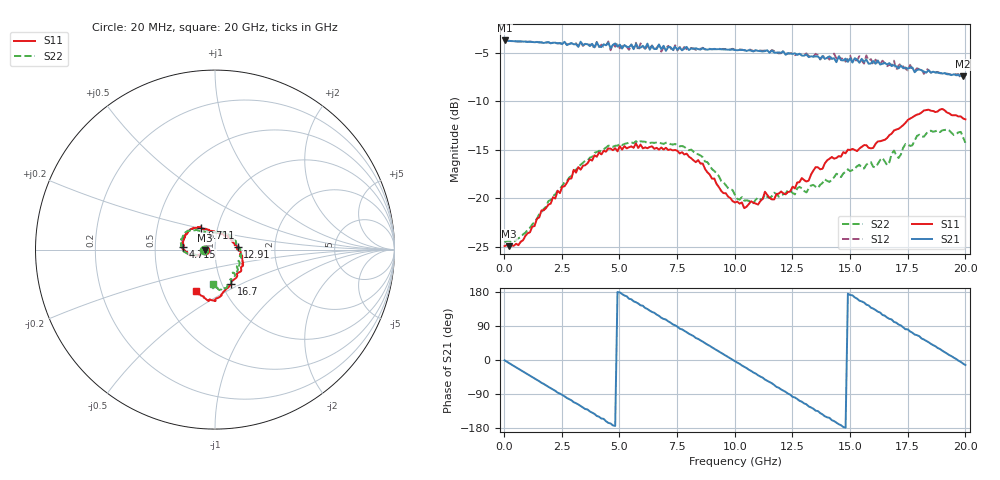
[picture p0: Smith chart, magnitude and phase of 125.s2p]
!Agilent Technologies,N5230A,US43500223,A.07.50.48
!Agilent N5230A: A.07.50.48
!Date: Saturday, October 10, 2015 18:30:05
!Correction: S11(Full 2 Port(1,2))
!S21(Full 2 Port(1,2))
!S12(Full 2 Port(1,2))
!S22(Full 2 Port(1,2))
!S2P File: Measurements: S11, S21, S12, S22:
# Hz S  RI  R 50
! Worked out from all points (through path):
!   201 points, 20 MHz to 20 GHz, reference 50 ohm
!   highest |S21| = -3.72 dB at 20 MHz (marker M1); lowest = -7.4 dB at 19.9 GHz (marker M2)
!   group delay of S21, straight-line fit = 102 ps
!   lowest |S11| = -24.9 dB at 219.8 MHz (marker M3), VSWR 1.12, Z = 44.6 - j0.157 ohm
!   |S11| at or under -10 dB: start of sweep to end of sweep
!   |S22| runs from -24.5 to -12.9 dB; largest |S21 - S12| = 0.048
!   S11 on the Smith chart (normalised r, x): 20 MHz: 0.89, -0.00; 4.715 GHz: 0.70, +0.02; 8.711 GHz: 0.84, +0.20; 12.91 GHz: 1.29, +0.04; 16.7 GHz: 1.11, -0.44; 20 GHz: 0.73, -0.36
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2e7  -0.0568 -3.59e-05  0.6516 -0.00899  0.6509 -0.00979  -0.0596 0.000289
2.198e8  -0.0567 -0.00175  0.6412 -0.0947  0.6414 -0.095  -0.0606 -0.00135
1.1189e9  -0.0645 -0.0179  0.4817 -0.4256  0.4813 -0.4244  -0.0684 -0.0178
1.9181e9  -0.0865 -0.034  0.21 -0.6041  0.2123 -0.601  -0.0928 -0.0281
2.6174e9  -0.1103 -0.0344  -0.0644 -0.6384  -0.0586 -0.6307  -0.1179 -0.029
3.4166e9  -0.1452 -0.0243  -0.3571 -0.5038  -0.3591 -0.494  -0.1506 -0.0241
4.7153e9  -0.1765 0.0166  -0.6133 -0.0805  -0.6202 -0.0896  -0.1845 0.0106
5.7143e9  -0.1839 0.0551  -0.553 0.2885  -0.5644 0.2884  -0.1907 0.05
6.7133e9  -0.1535 0.0906  -0.2783 0.5556  -0.2838 0.5481  -0.1773 0.0777
7.4126e9  -0.1358 0.1147  -0.0173 0.6047  -0.0269 0.6151  -0.1651 0.0958
8.7113e9  -0.0761 0.1196  0.4203 0.411  0.4146 0.4128  -0.112 0.1069
1.001e10  0.00722 0.095  0.5808 -0.0342  0.5823 -0.0217  -0.0382 0.0968
1.16084e10  0.0716 0.0681  0.2766 -0.5078  0.2886 -0.506  0.0364 0.096
1.29071e10  0.1263 0.0163  -0.1865 -0.5119  -0.1708 -0.5243  0.0831 0.0763
1.34066e10  0.1388 -0.00744  -0.3355 -0.4207  -0.31 -0.4385  0.1003 0.0611
1.43057e10  0.1528 -0.0489  -0.4998 -0.1706  -0.5192 -0.2028  0.1242 0.0328
1.5005e10  0.1569 -0.0835  -0.5212 0.0775  -0.5409 0.0558  0.138 -0.00867
1.59041e10  0.1225 -0.1334  -0.369 0.3319  -0.3901 0.3478  0.1415 -0.0599
1.67033e10  0.0904 -0.1915  -0.1585 0.4723  -0.176 0.4551  0.1217 -0.0939
1.83017e10  0.00358 -0.2854  0.2831 0.3427  0.2842 0.3706  0.0691 -0.2043
1.99001e10  -0.1038 -0.2362  0.4204 -0.0705  0.4259 -0.062  -0.0168 -0.206
2e10  -0.1079 -0.2317  0.4203 -0.0988  0.4288 -0.0792  -0.0131 -0.1933
